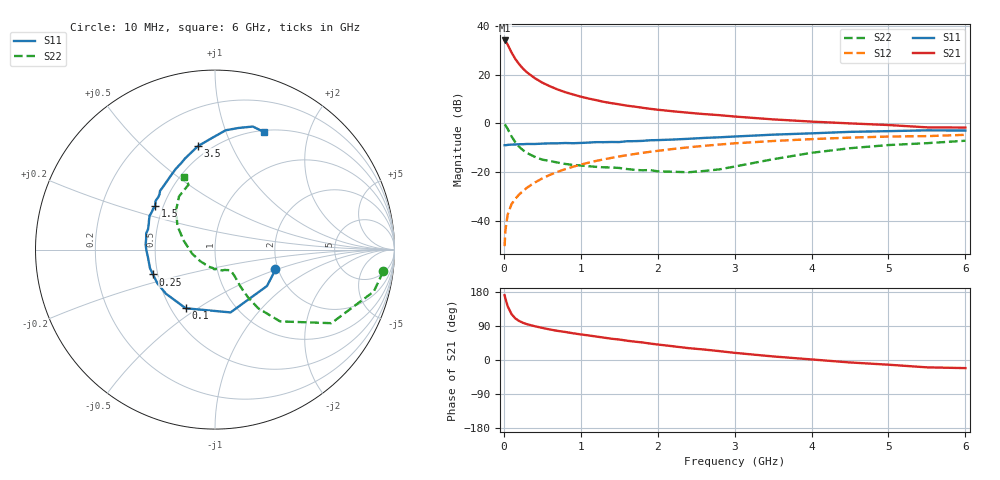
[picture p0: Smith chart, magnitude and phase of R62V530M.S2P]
! SIEMENS Small Signal Semiconductors
! BFR193
! Si NPN RF Bipolar Junction Transistor in SOT23
! VCE = 2.5 V  IC = 30 mA
! Common Emitter S-Parameters:  May  1996
# GHz  S  MA  R  50
!  f  S11  S21  S12  S22
! GHz  MAG  ANG  MAG  ANG  MAG  ANG  MAG  ANG
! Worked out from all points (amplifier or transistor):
!   36 points, 10 MHz to 6 GHz, reference 50 ohm
!   highest |S21| = 34.0 dB at 10 MHz (marker M1)
!   |S21| within 3 dB of that: start of sweep to 69.78 MHz
!   unconditionally stable (mu >= 1): 452.9 MHz to 1.877 GHz
!   at 250 MHz: K = 0.91, MSG = 25.1 dB, |S12| = -27.8 dB
!   at 1.4 GHz: K = 1.02, MAG = 10.3 dB, |S12| = -14.2 dB
!   at 6 GHz: K = 0.95, MSG = 1.5 dB, |S12| = -4.7 dB
!   lowest NFmin = 1.90 dB at 450 MHz
!   S11 on the Smith chart (normalised r, x): 10 MHz: 1.93, -0.49; 100 MHz: 0.59, -0.45; 250 MHz: 0.47, -0.15; 1.5 GHz: 0.45, +0.26; 3.5 GHz: 0.43, +0.75; 6 GHz: 0.52, +1.37
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0.01  0.3548 -18.2  50.27 171.0  0.003 82.0  0.9454 -7.4
0.02  0.3537 -35.0  48.94 162.4  0.0063 79.9  0.9149 -14.8
0.05  0.3605 -76.1  41.14 141.7  0.0134 69.4  0.767 -32.3
0.1  0.3654 -116.5  28.51 121.1  0.0219 65.9  0.54 -47.8
0.15  0.3676 -138.0  20.88 109.6  0.0283 66.0  0.406 -53.6
0.2  0.372 -149.7  16.28 102.8  0.0347 67.4  0.3277 -55.3
0.25  0.3722 -158.2  13.22 98.1  0.0406 69.2  0.2808 -55.5
0.3  0.3767 -164.2  11.14 94.5  0.0475 70.5  0.246 -55.4
0.4  0.3759 -173.3  8.505 89.2  0.0605 71.4  0.2059 -54.2
0.5  0.3825 -179.5  6.842 84.7  0.0739 71.7  0.1791 -53.4
0.6  0.3876 175.7  5.753 80.5  0.0876 71.7  0.1684 -53.3
0.7  0.3884 171.0  4.945 76.8  0.1009 71.1  0.1561 -53.4
0.9  0.3899 163.2  3.906 70.5  0.1284 69.2  0.1398 -55.3
1.1  0.4022 156.1  3.228 64.9  0.1553 67.0  0.1314 -60.3
1.3  0.4099 149.2  2.759 59.0  0.1821 64.5  0.1249 -64.7
1.5  0.4119 144.1  2.453 54.1  0.2086 61.9  0.1212 -72.3
1.9  0.4486 133.0  1.986 43.4  0.2596 56.3  0.1098 -92.5
2.2  0.4639 125.7  1.765 36.2  0.2972 51.8  0.1012 -110.6
3.5  0.5846 99.3  1.204 9.4  0.4334 31.5  0.183 163.5
4.5  0.6674 84.9  0.996 -6.5  0.5087 17.3  0.308 134.7
5.5  0.7174 72.9  0.826 -19.4  0.5455 3.3  0.3909 112.1
6  0.7095 67.2  0.818 -21.4  0.5803 -0.8  0.4388 113.5
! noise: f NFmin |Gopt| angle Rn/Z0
0.45  1.9  0.4  180  0.09
0.9  1.95  0.43  -173  0.11
1.8  2.4  0.58  -144  0.24
